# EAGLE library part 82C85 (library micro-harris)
MICROCONTROLLER/MEMORY DEVICE
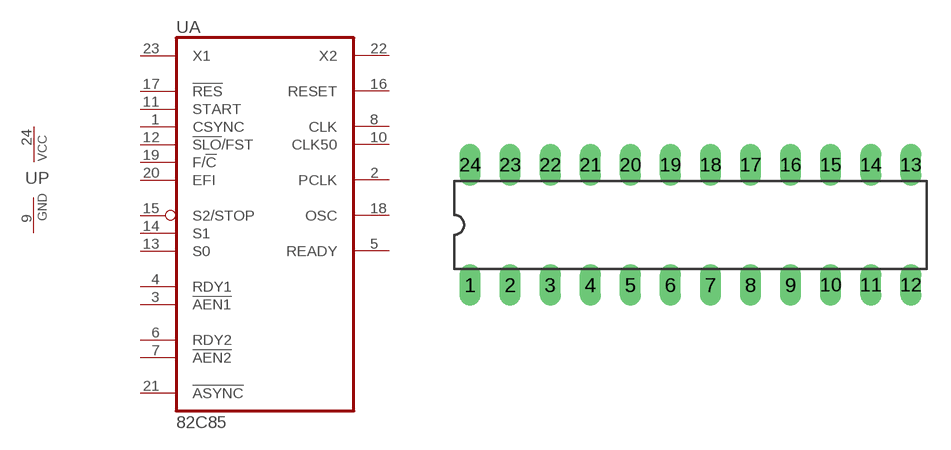
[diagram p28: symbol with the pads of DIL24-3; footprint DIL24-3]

Designator prefix U; gates A=82C85 P=PWRN

## 82C85 (OC_FARNELL: unknown; OC_NEWARK: unknown)  [DIL24-3]
1  A:CSYNC  in
2  A:PCLK  out
3  A:!AEN1  in
4  A:RDY1  in
5  A:READY  out
6  A:RDY2  in
7  A:!AEN2  in
8  A:CLK  out
9  P:GND  pwr
10  A:CLK50  out
11  A:START  in
12  A:!SLO!/FST  in
13  A:S0  in
14  A:S1  in
15  A:S2/STOP  in
16  A:RESET  out
17  A:!RES  in
18  A:OSC  out
19  A:F/!C  in
20  A:EFI  in
21  A:!ASYNC  in
22  A:X2  out
23  A:X1  in
24  P:VCC  pwr

## Footprint DIL24-3 (pad centres in mm)
Dual In Line Package 0.3 inch
drill 0.813 long: 1 -13.97,-3.81; 2 -11.43,-3.81; 3 -8.89,-3.81; 4 -6.35,-3.81; 5 -3.81,-3.81; 6 -1.27,-3.81; 7 1.27,-3.81; 8 3.81,-3.81; 9 6.35,-3.81; 10 8.89,-3.81; 11 11.43,-3.81; 12 13.97,-3.81; 13 13.97,3.81; 14 11.43,3.81; 15 8.89,3.81; 16 6.35,3.81; 17 3.81,3.81; 18 1.27,3.81; 19 -1.27,3.81; 20 -3.81,3.81; 21 -6.35,3.81; 22 -8.89,3.81; 23 -11.43,3.81; 24 -13.97,3.81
